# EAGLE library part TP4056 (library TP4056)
TP4056 Data sheet Dave.Calaway Eagle Library
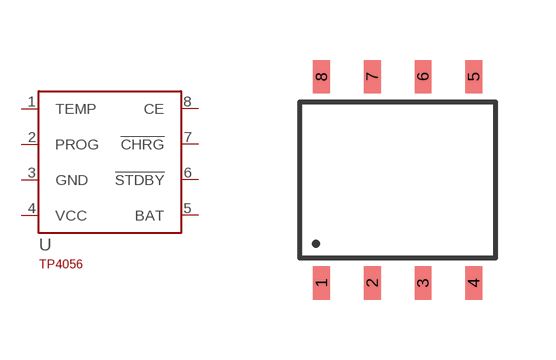
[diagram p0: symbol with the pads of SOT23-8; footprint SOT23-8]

Designator prefix -

## TP4056  [SOT23-8]
1  TEMP
2  PROG
3  GND
4  VCC
5  BAT
6  !STDBY
7  !CHRG
8  CE

## Footprint SOT23-8 (pad centres in mm)
Package SOP-8PP http://goo.gl/2DAeEi
smd 0.42 x 0.835: 1 -1.905,-2.58; 2 -0.635,-2.58; 3 0.635,-2.58; 4 1.905,-2.58; 5 1.905,2.58; 6 0.635,2.58; 7 -0.635,2.58; 8 -1.905,2.58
